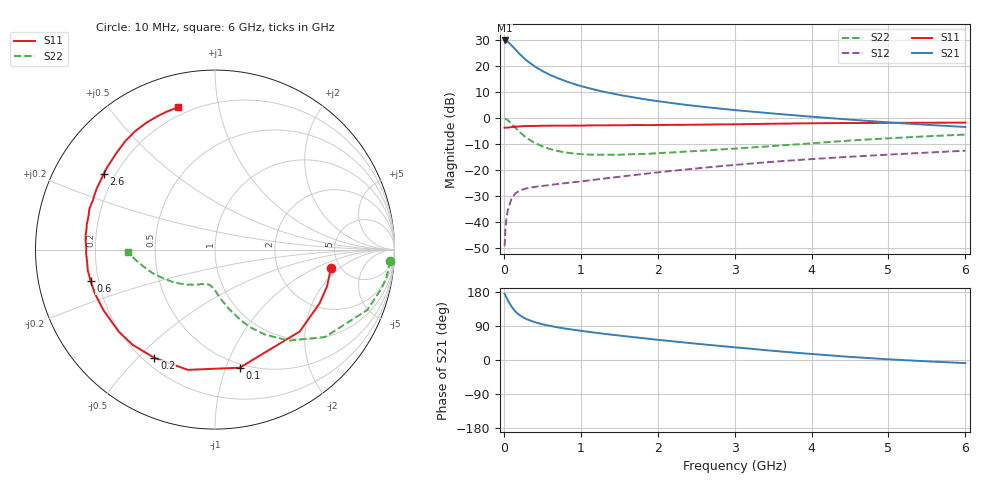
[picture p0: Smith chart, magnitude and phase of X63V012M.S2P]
! SIEMENS Small Signal Semiconductors
! BFP193W
! Si NPN RF Bipolar Junction Transistor in SOT343
! VCE = 3 V  IC = 12 mA
! Common Emitter S-Parameters:  April 1994
# GHz  S  MA  R  50
!  f  S11  S21  S12  S22
! GHz  MAG  ANG  MAG  ANG  MAG  ANG  MAG  ANG
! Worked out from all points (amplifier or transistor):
!   40 points, 10 MHz to 6 GHz, reference 50 ohm
!   highest |S21| = 29.8 dB at 10 MHz (marker M1)
!   |S21| within 3 dB of that: start of sweep to 136 MHz
!   unconditionally stable (mu >= 1): 1.212 GHz to 4.186 GHz
!   at 200 MHz: K = 0.25, MSG = 26.3 dB, |S12| = -27.9 dB
!   at 1.5 GHz: K = 1.09, MAG = 13.9 dB, |S12| = -22.5 dB
!   at 6 GHz: K = 0.93, MSG = 4.6 dB, |S12| = -12.5 dB
!   S11 on the Smith chart (normalised r, x): 10 MHz: 4.19, -1.53; 100 MHz: 0.47, -1.12; 200 MHz: 0.24, -0.56; 600 MHz: 0.17, -0.12; 2.6 GHz: 0.16, +0.30; 6 GHz: 0.16, +0.76
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0.01  0.6542 -9.2  30.82 174.6  0.0035 87.4  0.9777 -3.7
0.02  0.6571 -18.2  30.8 170.9  0.0072 81.9  0.9683 -9.1
0.03  0.655 -27.1  30.36 166.7  0.0105 79.4  0.9518 -13.3
0.05  0.6567 -44.0  29.13 158.2  0.0169 72.2  0.9129 -21.6
0.1  0.6722 -78.2  24.92 140.9  0.0286 56.9  0.7827 -38.5
0.15  0.6868 -102.7  20.71 128.0  0.0361 47.0  0.6531 -50.9
0.2  0.6912 -119.2  17.23 119.1  0.0403 41.3  0.5496 -59.5
0.25  0.7013 -130.8  14.65 112.6  0.043 37.3  0.4739 -65.8
0.3  0.7047 -139.4  12.58 107.5  0.0451 35.3  0.4124 -70.4
0.4  0.7073 -151.4  9.811 99.9  0.0479 33.3  0.335 -77.2
0.5  0.7126 -159.9  8.012 94.3  0.05 33.0  0.2866 -82.1
0.6  0.715 -165.8  6.743 89.9  0.0522 33.6  0.2549 -86.0
0.8  0.7159 -174.7  5.124 82.9  0.0567 36.3  0.22 -91.4
1.1  0.7227 176.2  3.773 74.4  0.0636 40.0  0.1996 -98.2
1.3  0.7248 170.9  3.199 69.2  0.0693 42.4  0.1982 -102.1
1.6  0.7305 164.3  2.626 62.2  0.078 45.0  0.2007 -107.2
2.2  0.7416 152.8  1.93 49.2  0.0976 47.6  0.2198 -117.9
2.6  0.7501 145.7  1.641 41.1  0.1118 48.0  0.2379 -125.1
3.2  0.7685 135.9  1.341 29.9  0.1339 46.9  0.2722 -135.9
4.5  0.8045 118.0  0.935 8.2  0.1814 41.1  0.3713 -159.2
5.5  0.8145 109.0  0.743 -3.5  0.2177 35.8  0.4476 -172.8
6  0.8192 104.6  0.676 -8.2  0.237 33.2  0.4834 -178.2
